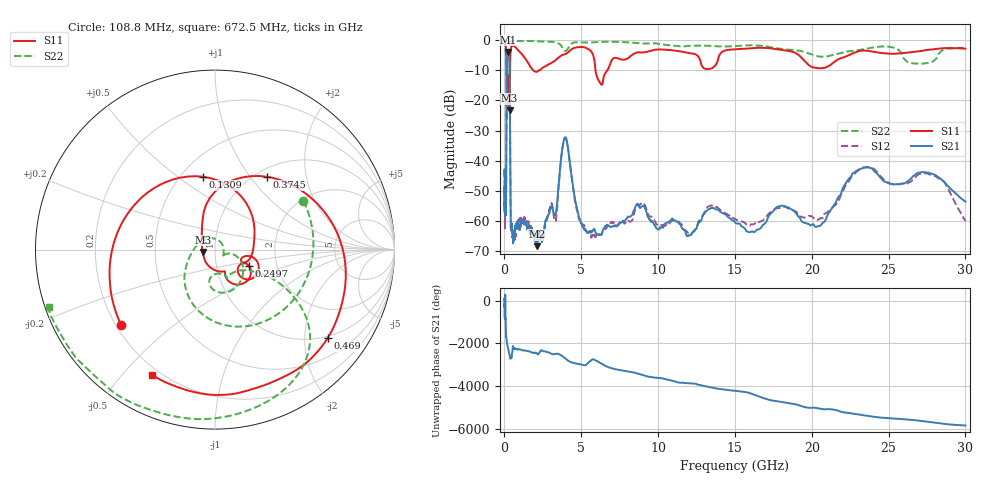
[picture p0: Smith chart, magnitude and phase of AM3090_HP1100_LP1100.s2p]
! Date/Time: Thu, Feb 28, 2019 2:07 PM
! Network Analyzer: Agilent Technologies E8364B Rev: A.07.50.67
! Sweep from 0.010 to 30.000 GHz, 1601 Points, Sweep Type: LOG
! Power Supply: 5.022 V, 0.002 A
# Hz S DB R 50
!freq MagS11 AngS11 MagS21 AngS21 MagS12 AngS12 MagS22 AngS22
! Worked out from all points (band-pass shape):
!   1601 points, 10 MHz to 30 GHz, reference 50 ohm
!   highest |S21| = -3.91 dB at 233.9 MHz (marker M1); lowest = -68.3 dB at 2.105 GHz (marker M2)
!   |S21| within 3 dB of the highest: 143.8 MHz to 324 MHz (180.2 MHz wide, 77 % of centre)
!   lowest |S11| = -23.2 dB at 333.7 MHz (marker M3), VSWR 1.15, Z = 43.6 - j1.18 ohm
!   |S11| at or under -10 dB: 136.1 MHz to 361.2 MHz (225.1 MHz wide, 90.5 % of centre); 1.867 GHz to 2.254 GHz (387.2 MHz wide, 18.8 % of centre); 5.926 GHz to 6.699 GHz (773.2 MHz wide, 12.2 % of centre)
!   |S22| runs from -26.4 to -0.1 dB; largest |S21 - S12| = 0.014
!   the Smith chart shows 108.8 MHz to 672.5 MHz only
!   S11 on the Smith chart (normalised r, x): 108.8 MHz: 0.22, -0.34; 130.9 MHz: 0.64, +0.62; 249.7 MHz: 1.43, -0.27; 374.5 MHz: 1.12, +1.21; 469 MHz: 0.96, -2.59; 672.5 MHz: 0.17, -0.60
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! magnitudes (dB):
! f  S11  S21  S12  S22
! 10 MHz  -0.2  -44.2  -45.4  -0.7
! 38.04 MHz  -0.4  -57.6  -55.2  -1.4
! 108.8 MHz  -3.5  -51.1  -52.3  -5.0
! 130.9 MHz  -7.7  -16.9  -16.9  -9.1
! 144.7 MHz  -13.0  -6.7  -6.6  -26.2
! 233.9 MHz  -15.8  -3.9  -3.9  -16.4
! 249.7 MHz  -13.7  -4.0  -4.0  -17.3
! 333.7 MHz  -23.2  -8.7  -8.6  -9.7
! 374.5 MHz  -6.1  -38.0  -37.7  -1.3
! 409.7 MHz  -3.1  -60.6  -59.4  -0.5
! 469 MHz  -2.0  -61.5  -62.2  -0.3
! 550.5 MHz  -1.9  -66.1  -64.1  -0.2
! 672.5 MHz  -2.2  -63.1  -65.0  -0.2
! 2.084 GHz  -10.5  -67.3  -63.8  -0.4
! 2.105 GHz  -10.5  -68.3  -63.8  -0.4
! 3.335 GHz  -6.6  -57.7  -60.1  -0.8
! 3.953 GHz  -4.7  -32.3  -32.3  -3.6
! 5.18 GHz  -2.4  -62.7  -61.3  -0.8
! 7.926 GHz  -6.3  -59.3  -60.0  -0.7
! 20.1 GHz  -9.1  -61.0  -59.0  -4.9
! 23.48 GHz  -3.5  -42.3  -42.2  -2.9
! 30 GHz  -2.8  -53.5  -60.0  -2.6
